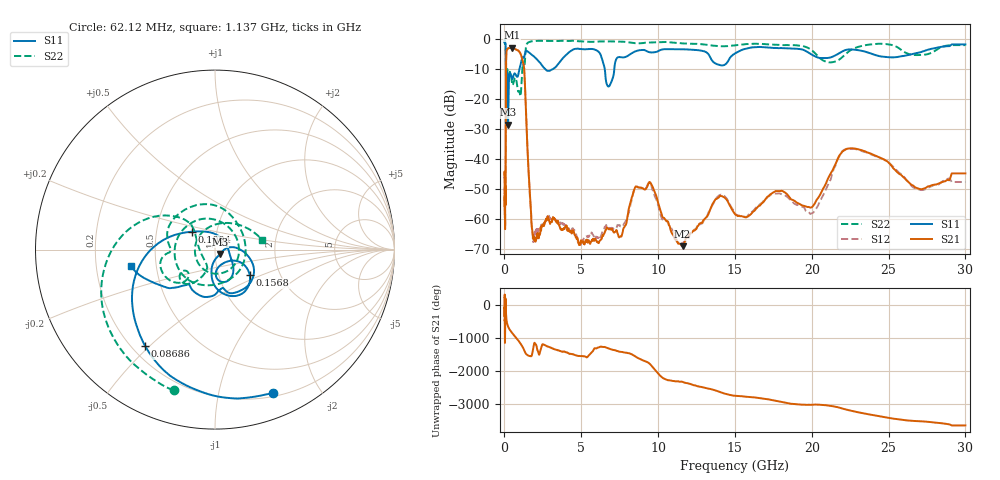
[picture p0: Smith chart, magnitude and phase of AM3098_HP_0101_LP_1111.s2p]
! Date/Time: Thu, Feb 28, 2019 8:37 AM
! Network Analyzer: Agilent Technologies E8364B Rev: A.07.50.67
! Sweep from 0.010 to 30.000 GHz, 1601 Points, Sweep Type: LOG
! Power Supply: 5.022 V, 0.002 A
# Hz S DB R 50
!freq MagS11 AngS11 MagS21 AngS21 MagS12 AngS12 MagS22 AngS22
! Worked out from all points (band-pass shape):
!   1601 points, 10 MHz to 30 GHz, reference 50 ohm
!   highest |S21| = -2.76 dB at 498 MHz (marker M1); lowest = -69.2 dB at 11.59 GHz (marker M2)
!   |S21| within 3 dB of the highest: 115 MHz to 1.113 GHz (998 MHz wide, 163 % of centre)
!   lowest |S11| = -28.6 dB at 235.1 MHz (marker M3), VSWR 1.08, Z = 52.8 - j2.65 ohm
!   |S11| at or under -10 dB: 97.47 MHz to 973 MHz (875.5 MHz wide, 164 % of centre); 2.669 GHz to 3.136 GHz (467.1 MHz wide, 16.1 % of centre); 6.528 GHz to 7.149 GHz (621.1 MHz wide, 9.08 % of centre)
!   |S22| runs from -22.1 to -0.5 dB; largest |S21 - S12| = 0.01
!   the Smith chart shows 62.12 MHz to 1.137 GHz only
!   S11 on the Smith chart (normalised r, x): 62.12 MHz: 0.23, -1.46; 86.86 MHz: 0.25, -0.48; 100.4 MHz: 0.76, +0.16; 156.8 MHz: 1.41, -0.42; 1.137 GHz: 0.36, -0.09
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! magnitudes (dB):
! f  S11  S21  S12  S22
! 10 MHz  -0.3  -45.2  -46.6  -0.6
! 38.04 MHz  -0.5  -58.9  -60.2  -1.0
! 62.12 MHz  -1.3  -51.3  -52.3  -1.7
! 86.86 MHz  -3.6  -40.4  -40.2  -3.9
! 100.4 MHz  -15.8  -13.3  -13.3  -19.8
! 144.7 MHz  -17.3  -3.7  -3.7  -13.7
! 156.8 MHz  -12.4  -3.6  -3.5  -11.6
! 235.1 MHz  -28.6  -2.9  -2.9  -11.9
! 309.6 MHz  -12.6  -2.9  -2.8  -11.2
! 498 MHz  -13.2  -2.8  -2.7  -15.0
! 550.5 MHz  -12.7  -2.9  -2.9  -15.1
! 1.137 GHz  -6.4  -6.2  -6.2  -11.4
! 1.308 GHz  -5.4  -12.2  -12.1  -8.9
! 1.82 GHz  -5.3  -64.4  -65.4  -0.6
! 2.084 GHz  -6.5  -66.6  -63.5  -0.5
! 7.926 GHz  -5.8  -61.7  -60.6  -0.9
! 9.396 GHz  -4.2  -48.1  -47.8  -1.0
! 11.59 GHz  -3.3  -69.2  -68.3  -1.3
! 14.02 GHz  -8.6  -52.3  -52.0  -2.3
! 19.9 GHz  -4.8  -56.3  -58.4  -3.3
! 22.67 GHz  -3.4  -36.4  -36.7  -3.2
! 30 GHz  -1.7  -44.8  -47.7  -1.9
